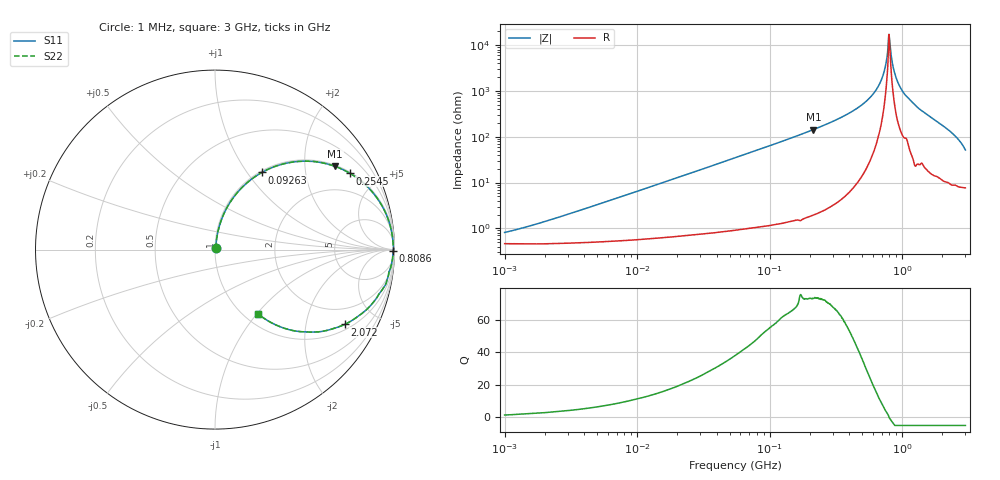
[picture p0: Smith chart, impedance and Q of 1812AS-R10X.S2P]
!s-Parameter Generated by FASTRON Sdn. Bhd.
!FASTRON P/N : 1812AS-R10X
!Keysight Technologies,E4991B,MY54100416,A.01.15
!Date created: Fri Oct 13 14:44:38 2023
!Version  : Rev00 Fri Oct 13 14:44:38 2023
!Data & Calibration Information:
!Freq	S11	S21	S12	S22
!PortZ  Port1:50+j0  Port2:50+j0
!When reading, reference impedance value at option line is always used.
! Remarks : This data is being provided solely for informational purposes.
# Hz S dB R 50
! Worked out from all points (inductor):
!   1601 points, 1 MHz to 3 GHz, reference 50 ohm
!   read as one part in series: L = 105 nH near 2.097 MHz
!   highest Q = 73.4 at 213.6 MHz (marker M1), where L = 107 nH
!   self-resonance near 796.6 MHz
!   S11 on the Smith chart (normalised r, x): 1 MHz: 1.01, +0.01; 92.63 MHz: 1.02, +1.18; 254.5 MHz: 1.05, +3.52; 808.6 MHz: open; 2.072 GHz: 1.21, -3.32; 3 GHz: 1.15, -1.02
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1000000  -41.83 54.9  -0.04 -0.4  -0.04 -0.4  -41.83 54.9
3804036  -31.96 77.5  -0.04 -1.4  -0.04 -1.4  -31.96 77.5
1.447069e7  -20.77 80.9  -0.09 -5.2  -0.09 -5.2  -20.77 80.9
5.477226e7  -9.78 69.6  -0.56 -18.9  -0.56 -18.9  -9.78 69.6
9.262894e7  -5.98 58.8  -1.36 -30.2  -1.36 -30.2  -5.98 58.8
2.083556e8  -1.86 35.4  -4.73 -53.8  -4.73 -53.8  -1.86 35.4
2.136344e8  -1.78 34.7  -4.90 -54.5  -4.90 -54.5  -1.78 34.7
2.545267e8  -1.27 29.4  -6.18 -59.8  -6.18 -59.8  -1.27 29.4
4.219165e8  -0.37 15.4  -11.51 -73.4  -11.51 -73.4  -0.37 15.4
5.899715e8  -0.12 7.2  -18.08 -80.2  -18.08 -80.2  -0.12 7.2
7.064253e8  -0.07 2.9  -25.81 -79.9  -25.81 -79.9  -0.07 2.9
7.38967e8  -0.06 1.9  -29.58 -76.7  -29.58 -76.7  -0.06 1.9
7.730077e8  -0.06 0.8  -35.97 -66.1  -35.97 -66.1  -0.06 0.8
7.925923e8  -0.05 0.1  -44.69 -25.5  -44.69 -25.5  -0.05 0.1
8.086166e8  -0.06 -0.4  -40.60 41.8  -40.60 41.8  -0.06 -0.4
8.543737e8  -0.07 -1.6  -30.59 72.7  -30.59 72.7  -0.07 -1.6
8.892696e8  -0.08 -2.6  -26.76 77.3  -26.76 77.3  -0.08 -2.6
1.023018e9  -0.15 -6.1  -19.42 77.7  -19.42 77.7  -0.15 -6.1
1.327057e9  -0.36 -13.2  -12.80 73.4  -12.80 73.4  -0.36 -13.2
2.071593e9  -1.58 -30.0  -6.00 56.3  -6.00 56.3  -1.58 -30.0
2.568929e9  -3.49 -43.2  -3.26 41.8  -3.26 41.8  -3.49 -43.2
3e9  -7.30 -56.2  -1.52 25.3  -1.52 25.3  -7.30 -56.2
